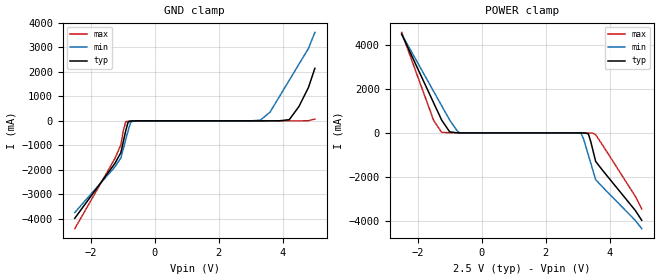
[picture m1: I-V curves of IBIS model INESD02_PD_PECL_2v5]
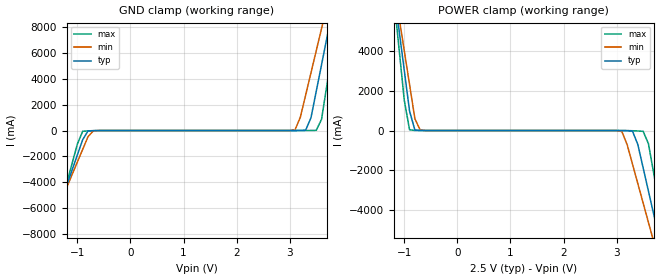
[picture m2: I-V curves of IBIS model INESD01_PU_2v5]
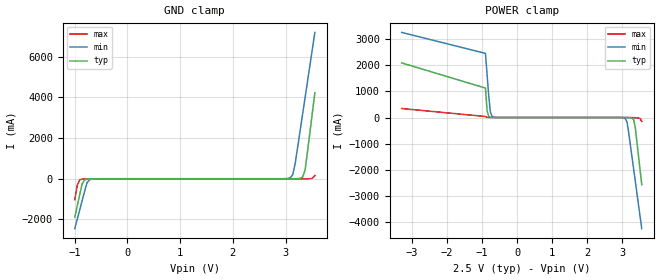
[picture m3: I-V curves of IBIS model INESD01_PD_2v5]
|   This file is an IBIS representation of the   |
|   Integrated Device Technology, Inc.   |
|   ICS8761I   |
|   LOW VOLTAGE, LOW SKEW,PCI / PCI-X CLOCK GENERATOR   |
[IBIS Ver]   4.1
[File name]   8761i.ibs
[File Rev]   2.0
[Date]   22 Jun 2009 | Last modified
|   Oct 14 2002 | Generated
[Source]   Originated at Integrated Device Technology, Inc.
[Disclaimer]
IDT hereby grants the user of this IBIS model a non-exclusive,
nontransferable license to use this IBIS model under the following terms.
Before using this IBIS model, the user should read this license.
If the user does not accept these terms,  the IBIS model should be
returned to IDT within 30 days.
   The user is granted this license only to use the IBIS model and
is not granted rights to sell, load, rent, lease or license the IBIS
model in whole or in part, or in modified form to anyone other than
user. User may modify the IBIS model to suit its specific
applications but rights to derivative works and such modifications
shall belong to IDT.
   This IBIS model is provided on an "AS IS" basis and IDT makes
absolutely no warranty with respect to the information contained
herein. IDT DISCLAIMS AND CUSTOMER WAIVES ALL WARRANTIES, EXPRESS
OR IMPLIED, INCLUDING WARRANTIES OF MERCHANTABILITY OR FITNESS FOR
A PARTICULAR PURPOSE. The entire risk as to quality and performance
is with the Customer. ACCORDINGLY, IN NO EVENT SHALL THE COMPANY BE
LIABLE FOR ANY DAMAGES, WHETHER IN CONTRACT OR TORT,INCLUDING ANY
LOST PROFITS OR OTHER INCIDENTAL, CONSEQUENTIAL, EXEMPLARY, OR
PUNITIVE DAMAGES ARISING OUT OF THE USE OR APPLICATION OF THE IBIS
model provided in this package. Further, IDT reserves the right to
make changes without notice to any product herein to improve
reliability, function, or design. IDT does not convey any license
under patent rights or any other intellectual property rights,
including those of third parties.
   IDT is not obligated to provide maintenance or support
for the licensed IBIS model.
[Copyright]   Copyright 2002 by Integrated Device Technology, Inc.
[Component]   ICS8761I
[Manufacturer] Integrated Device Technology, Inc.
[Package]
|LQFP
|lead + wire
|   typ   min   max
R_pkg   25.91068767m   19.86813682m   35.470595m
L_pkg   0.200540749n   0.041634089n   0.451946652n
C_pkg   0.055023162p   0.043398018p   0.073415279p
[Pin] signal_name   model_name   R_pin   L_pin   C_pin
1   REF_CLK   INESD02_PD_PECL   33.00322952m  0.387060014n   0.068668363p
2   GND   GND   30.31815532m  0.316448084n   0.063502602p
3   XTAL1   NC   27.70565070m  0.247744585n   0.058476456p
4   XTAL2   NC   25.38342437m  0.186674809n   0.054008771p
5   VDD   POWER   23.35147632m  0.133238754n   0.050099546p
6   XTAL_SEL   INESD01_PU   22.69835017m  0.116062879n   0.048843010p
7   PLL_SEL   INESD01_PU   22.19036316m  0.102703866n   0.047865704p
8   VDDA   POWER   19.86813682m  0.041634089n   0.043398018p
9   VDD   POWER   21.53723700m  0.085527991n   0.046609167p
10   D_SELC0   INESD01_PU   22.19036316m  0.102703866n   0.047865704p
11   D_SELC1   INESD01_PU   21.68237615m  0.089344852n   0.046888398p
12   OEC   INESD01_PU   22.62578059m  0.114154449n   0.048703395p
13   OEA   INESD01_PU   25.38342437m  0.186674809n   0.054008771p
14   D_SELA0   INESD01_PD   27.77822027m  0.249653016n   0.058616071p
15   D_SELA1   INESD01_PD   29.66502917m  0.299272210n   0.062246066p
16   GND   GND   31.11642063m  0.337440820n   0.065038369p
17   GND   GND   35.47059500m  0.451946652n   0.073415279p
18   QA0   COUT10_15_OHM   32.78552080m  0.381334722n   0.068249518p
19   VDDOA   POWER   30.17301618m  0.312631223n   0.063223372p
20   QA1   COUT10_15_OHM   27.85078985m  0.251561447n   0.058755687p
21   GND   GND   24.80286778m  0.171407364n   0.052891850p
22   QA2   COUT10_15_OHM   23.27890675m  0.131330323n   0.049959931p
23   VDDOA   POWER   21.97265444m  0.096978574n   0.047446858p
24   QA3   COUT10_15_OHM   21.53723700m  0.085527991n   0.046609167p
25   GND   GND   20.73897170m  0.064535255n   0.045073400p
26   QB0   COUT10_15_OHM   21.82751529m  0.093161713n   0.047167628p
27   VDDOB   POWER   22.48064145m  0.110337588n   0.048424164p
28   QB1   COUT10_15_OHM   23.35147632m  0.133238754n   0.050099546p
29   GND   GND   25.38342437m  0.186674809n   0.054008771p
30   QB2   COUT10_15_OHM   27.77822027m  0.249653016n   0.058616071p
31   VDDOB   POWER   30.31815532m  0.316448084n   0.063502602p
32   QB3   COUT10_15_OHM   32.05982507m  0.362250417n   0.066853366p
33   GND   GND   31.11642063m  0.337440820n   0.065038369p
34   D_SELB1   INESD01_PD   29.66502917m  0.299272210n   0.062246066p
35   D_SELB0   INESD01_PD   27.77822027m  0.249653016n   0.058616071p
36   OEB   INESD01_PU   25.45599394m  0.188583239n   0.054148386p
37   OED   INESD01_PU   22.62578059m  0.114154449n   0.048703395p
38   D_SELD1   INESD01_PD   21.75494572m  0.091253282n   0.047028013p
39   D_SELD0   INESD01_PD   22.19036316m  0.102703866n   0.047865704p
40   VDD   POWER   21.53723700m  0.085527991n   0.046609167p
41   MR   INESD01_PD   19.94070640m  0.043542519n   0.043537634p
42   FBDIV_SEL1   INESD01_PU   22.19036316m  0.102703866n   0.047865704p
43   FBDIV_SEL0   INESD01_PD   22.69835017m  0.116062879n   0.048843010p
44   VDD   POWER   23.35147632m  0.133238754n   0.050099546p
45   FB_IN   INESD02_PD_PECL   25.38342437m  0.186674809n   0.054008771p
46   VDDOFB   POWER   27.77822027m  0.249653016n   0.058616071p
47   FB_OUT   COUT10_15_OHM   30.31815532m  0.316448084n   0.063502602p
48   GND   GND   33.07579910m  0.388968444n   0.068807978p
49   QD3   COUT10_15_OHM   33.07579910m  0.388968444n   0.068807978p
50   VDDOD   POWER   30.31815532m  0.316448084n   0.063502602p
51   QD2   COUT10_15_OHM   27.77822027m  0.249653016n   0.058616071p
52   GND   GND   25.38342437m  0.186674809n   0.054008771p
53   QD1   COUT10_15_OHM   23.35147632m  0.133238754n   0.050099546p
54   VDDOD   POWER   22.48064145m  0.110337588n   0.048424164p
55   QD0   COUT10_15_OHM   21.82751529m  0.093161713n   0.047167628p
56   GND   GND   20.73897170m  0.064535255n   0.045073400p
57   QC3   COUT10_15_OHM   21.53723700m  0.085527991n   0.046609167p
58   VDDOC   POWER   22.19036316m  0.102703866n   0.047865704p
59   QC2   COUT10_15_OHM   23.27890675m  0.131330323n   0.049959931p
60   GND   GND   24.80286778m  0.171407364n   0.052891850p
61   QC1   COUT10_15_OHM   27.85078985m  0.251561447n   0.058755687p
62   VDDOC   POWER   30.24558575m  0.314539654n   0.063362987p
63   QC0   COUT10_15_OHM   32.78552080m  0.381334722n   0.068249518p
64   GND   GND   35.47059500m  0.451946652n   0.073415279p
[Model Selector] INESD02_PD_PECL
INESD02_PD_PECL_2v5  Buffer selection for 2v5
INESD02_PD_PECL_3v3  Buffer selection for 3v3
[Model Selector] INESD01_PU
INESD01_PU_2v5  Buffer selection for 2v5
INESD01_PU_3v3  Buffer selection for 3v3
[Model Selector] INESD01_PD
INESD01_PD_2v5  Buffer selection for 2v5
INESD01_PD_3v3  Buffer selection for 3v3
[Model Selector] COUT10_15_OHM
COUT10_15_OHM_2v5  Buffer selection for 2v5
COUT10_15_OHM_3v3  Buffer selection for 3v3
| Models and submodels in the file (8): INESD02_PD_PECL_2v5 (Input), INESD01_PU_2v5 (Input), INESD01_PD_2v5 (Input), COUT10_15_OHM_2v5 (Output), INESD02_PD_PECL_3v3 (Input), INESD01_PU_3v3 (Input), INESD01_PD_3v3 (Input), COUT10_15_OHM_3v3 (Output)
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[Model] INESD02_PD_PECL_2v5
Model_type   Input
Polarity   Non-Inverting
Vinl = 0.8V
Vinh = 2.0V
|   typ   min   max
C_comp   2pF   1.5pF   2.5pF
|   typ   min   max
[Voltage range]  2.5V   2.375V   2.625V
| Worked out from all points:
|   GND clamp passes 1 mA (typ) near -0.59 V on its own axis
|   POWER clamp passes 1 mA (typ) near -0.69 V on its own axis
[GND_clamp]
|Voltage   I(typ)   I(min)   I(max)
-2.5V     -3.983A    -3.749A    -4.408A
-1.25V    -1.747A    -1.889A    -1.551A
-1.061V   -1.3A      -1.517A    -979.1mA
-909.1mV  -407.1mA   -774.3mA   -35.24mA
-833.3mV  -48.47mA   -403.4mA   -14.47mA
-757.6mV  -7.272mA   -70.21mA   -9.677mA
-681.8mV  -2.863mA   -7.067mA   -5.73mA
3.3V      167.2uA    32.81mA    49.66uA
3.6V      586.4uA    357.8mA    70.1uA
4.2V      47.81mA    1.661A     649.6uA
4.8V      1.366A     2.965A     5.596mA
5V        2.15A      3.618A     75.79mA
[POWER_clamp]
|Voltage   I(typ)   I(min)   I(max)
-2.5V     4.503A     4.499A     4.579A
-1.5V     1.366A     1.889A     566.5mA
-1.25V    582.4mA    1.237A     24.21mA
-1V       47.81mA    585.7mA    3.595mA
-681.8mV  586.4uA    6.896mA    416.8uA
3.03V     -323.1uA   -3.378mA   -47.98uA
3.106V    -1.127mA   -30.71mA   -286.5uA
3.182V    -2.863mA   -273.7mA   -1.276mA
3.333V    -48.47mA   -1.016A    -7.036mA
3.561V    -1.3A      -2.13A     -81.94mA
4.8V      -3.536A    -3.991A    -2.894A
5V        -3.983A    -4.363A    -3.465A
[Model] INESD01_PU_2v5
Model_type   Input
Polarity   Non-Inverting
Vinl = 1.4V
Vinh = 1.85V
|   typ   min   max
C_comp   2pF   1.5pF   2.5pF
|   typ   min   max
[Voltage range]  2.5V   2.375V   2.625V
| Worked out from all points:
|   GND clamp passes 1 mA (typ) near -0.54 V on its own axis
|   POWER clamp passes 1 mA (typ) near -0.66 V on its own axis
[GND_clamp]
|Voltage   I(typ)   I(min)   I(max)
-2.5V     -19.6A     -17.18A    -23.67A
-1.6V     -8.969A    -8.332A    -10.1A
-1.5V     -7.788A    -7.349A    -8.588A
-900mV    -707.1mA   -1.46A     -57.43mA
-700mV    -7.027mA   -24.05mA   -13.28mA
3.1V      199.2uA    53.94mA    11.78uA
3.3V      28.4mA     2.748A     652.4uA
3.5V      3.045A     6.192A     15.72mA
3.6V      5.115A     7.914A     872.4mA
3.7V      7.185A     9.638A     3.52A
3.9V      11.33A     13.09A     8.818A
5V        34.14A     32.07A     37.99A
[POWER_clamp]
|Voltage   I(typ)   I(min)   I(max)
-1.5V     9.257A     9.207A     9.48A
-1.2V     7.185A     7.484A     6.83A
-1.1V     5.115A     5.761A     4.182A
-900mV    976.9mA    2.318A     34.23mA
-700mV    1.582mA    24.31mA    1.044mA
3.1V      -2.107mA   -51.03mA   -534.5uA
3.3V      -35.62mA   -1.705A    -10.86mA
3.5V      -1.886A    -3.666A    -39.41mA
3.6V      -3.066A    -4.647A    -666.9mA
3.8V      -5.426A    -6.612A    -3.684A
3.9V      -6.607A    -7.595A    -5.193A
5V        -19.6A     -18.41A    -21.79A
[Model] INESD01_PD_2v5
Model_type   Input
Polarity   Non-Inverting
Vinl = 0.8V
Vinh = 2.0V
|   typ   min   max
C_comp   2pF   1.5pF   2.5pF
|   typ   min   max
[Voltage range]  2.5V   2.375V   2.625V
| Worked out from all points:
|   GND clamp passes 1 mA (typ) near -0.55 V on its own axis
|   POWER clamp passes 1 mA (typ) near -0.68 V on its own axis
[GND_clamp]
|Voltage I(typ)   I(min)   I(max)
-1V       -1.886A    -2.451A    -1.028A
-953.5mV  -1.338A    -1.994A    -328mA
-907mV    -789.6mA   -1.537A    -53.04mA
-860.5mV  -251.4mA   -1.081A    -21.51mA
-767.5mV  -17.28mA   -198.8mA   -10.01mA
-674.5mV  -5.28mA    -15.38mA   -3.684mA
3.092V    224.5uA    49.06mA    51.52uA
3.139V    500.8uA    208.3mA    52.98uA
3.185V    1.252mA    774.6mA    56.66uA
3.325V    81.55mA    3.177A     200uA
3.371V    416.9mA    3.978A     464.6uA
3.557V    4.225A     7.185A     159.2mA
[POWER_clamp]
|Voltage   I(typ)   I(min)   I(max)
-3.3V     2.083A     3.246A     343.1mA
-907mV    1.122A     2.445A     37.78mA
-860.5mV  267.5mA    1.644A     5.973mA
-814mV    47.03mA    844mA      1.727mA
-767.5mV  9.66mA     215.3mA    677uA
-674.5mV  960.6uA    12.66mA    131.4uA
3.092V    -1.849mA   -49.09mA   -51.51uA
3.139V    -3.491mA   -186mA     -159.7uA
3.325V    -84.03mA   -1.955A    -5.102mA
3.371V    -365.4mA   -2.411A    -8.31mA
3.51V     -2.01A     -3.782A    -35.44mA
3.557V    -2.558A    -4.239A    -152.3mA
